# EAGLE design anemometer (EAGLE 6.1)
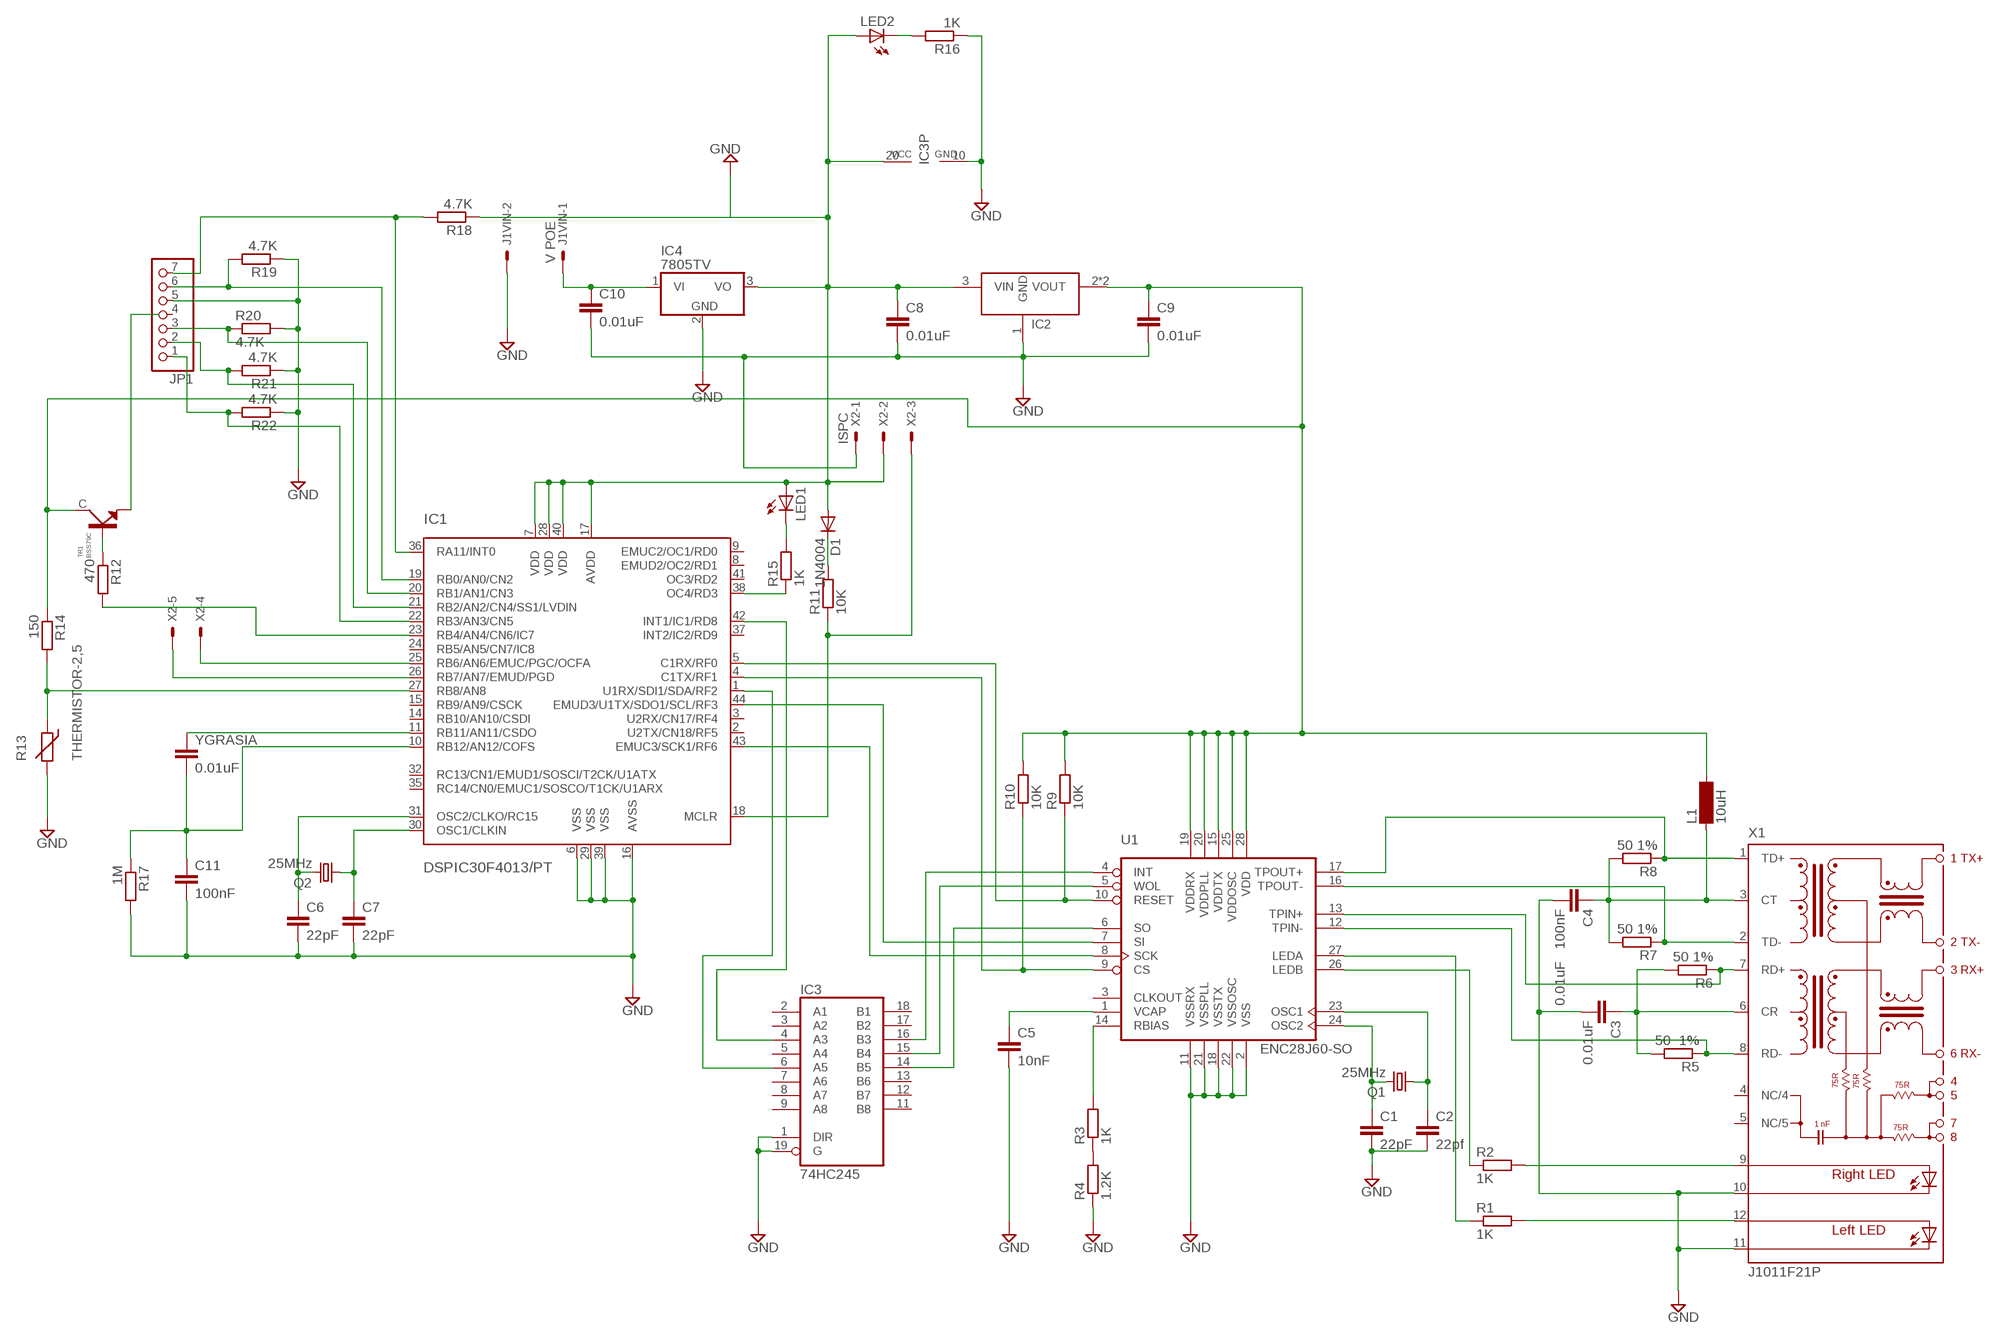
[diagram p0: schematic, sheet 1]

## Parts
C1  22pF  C-EUC0805  [C0805]
C2  22pf  C-EUC0805  [C0805]
C3  0.01uF  C-EUC0805  [C0805]
C4  0.01uF 100nF  C-EUC0805  [C0805]
C5  10nF  C-EU050-025X075  [C050-025X075]
C6  22pF  C-EUC0805  [C0805]
C7  22pF  C-EUC0805  [C0805]
C8  0.01uF  C-EU050-024X044  [C050-024X044]
C9  0.01uF  C-EU050-024X044  [C050-024X044]
C10  0.01uF  C-EU050-024X044  [C050-024X044]
C11  100nF  C-EUC0805  [C0805]
D1  1N4004  [DO41-10]
IC1  DSPIC30F4013/PT  [TQFP44]
IC2  TC2117-3.3  [SOT-223]
IC3  74HC245  [TSSOP20]
IC4  7805TV  [TO220V]
J1VIN  V POE  22-27-2021-02  [6410-02]
JP1  PINHD-1X7  [1X07]
L1  10uH  SM-1206  [SM-1206]
LED1  LEDSML0805  [SML0805]
LED2  LEDSML0805  [SML0805]
Q1  25MHz  CRYSTALHC49S  [HC49/S]
Q2  25MHz  CRYSTALHC49S  [HC49/S]
R1  1K  R-EU_R0805W  [R0805W]
R2  1K  R-EU_R0805W  [R0805W]
R3  1K  R-EU_R0805W  [R0805W]
R4  1.2K  R-EU_R0805W  [R0805W]
R5  50 1%  R-EU_R0603  [R0603]
R6  50 1%  R-EU_R0603  [R0603]
R7  50 1%  R-EU_R0603  [R0603]
R8  50 1%  R-EU_R0603  [R0603]
R9  10K  R-EU_R0805W  [R0805W]
R10  10K  R-EU_R0805W  [R0805W]
R11  10K  R-EU_R0805W  [R0805W]
R12  470  R-EU_R0805W  [R0805W]
R13  THERMISTOR-2,5  [RS-2,5]
R14  150  R-EU_R0805W  [R0805W]
R15  1K  R-EU_R0805W  [R0805W]
R16  1K  R-EU_R0805W  [R0805W]
R17  1M  R-EU_R0805W  [R0805W]
R18  4.7K  R-EU_R0805W  [R0805W]
R19  4.7K  R-EU_R0805W  [R0805W]
R20  4.7K  R-EU_R0805W  [R0805W]
R21  4.7K  R-EU_R0805W  [R0805W]
R22  4.7K  R-EU_R0805W  [R0805W]
TR1  BSS79C  [SOT23-EBC]
U1  ENC28J60-SO  [SO28W]
X1  J1011F21P  [J1]
X2  ISPC  22-23-2051  [22-23-2051]
YGRASIA  0.01uF  C-EU050-024X044  [C050-024X044]

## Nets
GND: C1.2 C2.2 C3.2 C4.2 C5.2 C6.2 C7.2 C8.2 C9.2 C10.2 C11.2 IC1.6(VSS) IC1.16(AVSS) IC1.29(VSS) IC1.39(VSS) IC2.1(GND) IC3.1(DIR) IC3.10(GND) IC3.19(G) IC4.2(GND) J1VIN.2 JP1.5 R4.1 R13.2 R16.1 R17.2 R19.1 R20.2 R21.1 R22.1 U1.2(VSS) U1.11(VSSRX) U1.18(VSSTX) U1.21(VSSPLL) U1.22(VSSOSC) X1.10(C-R) X1.11(C-L) X2.1
N$1: C1.1 Q1.2 U1.24(OSC2)
N$2: C2.1 Q1.1 U1.23(OSC1)
N$3: R1.1 U1.27(LEDA)
N$4: R1.2 X1.12(AL)
N$5: R2.1 U1.26(LEDB)
N$6: R2.2 X1.9(A-R)
N$7: R3.1 R4.2
N$8: R3.2 U1.14(RBIAS)
N$9: R6.1 U1.13(TPIN+) X1.7(RD+)
N$10: R5.1 U1.12(TPIN-) X1.8(RD-)
N$11: C3.1 R5.2 R6.2 X1.6(CR)
N$12: C6.1 IC1.31(OSC2/CLKO/RC15) Q2.2
N$13: R7.1 U1.16(TPOUT-) X1.2(TD-)
N$14: R8.1 U1.17(TPOUT+) X1.1(TD+)
N$15: C4.1 L1.1 R7.2 R8.2 X1.3(CT)
N$16: C7.1 IC1.30(OSC1/CLKIN) Q2.1
N$17: C5.1 U1.1(VCAP)
N$18: IC1.5(C1RX/RF0) R9.1 U1.10(RESET)
N$19: IC1.4(C1TX/RF1) R10.1 U1.9(CS)
N$20: IC1.18(MCLR) R11.1 X2.3
N$21: C10.1 IC4.1(VI) J1VIN.1
N$22: D1.C R11.2
N$23: C9.1 IC2.2(VOUT) IC2.4(VOUT) L1.2 R9.2 R10.2 R14.1 TR1.C U1.15(VDDTX) U1.19(VDDRX) U1.20(VDDPLL) U1.25(VDDOSC) U1.28(VDD)
N$24: IC3.14(B5) U1.6(SO)
N$25: C8.1 D1.A IC1.7(VDD) IC1.17(AVDD) IC1.28(VDD) IC1.40(VDD) IC2.3(VIN) IC3.20(VCC) IC4.3(VO) LED1.A LED2.A R18.1 X2.2
N$26: IC3.15(B4) U1.5(WOL)
N$27: IC3.16(B3) U1.4(INT)
N$28: IC1.26(RB7/AN7/EMUD/PGD) X2.5
N$29: IC1.25(RB6/AN6/EMUC/PGC/OCFA) X2.4
N$30: IC1.1(U1RX/SDI1/SDA/RF2) IC3.6(A5)
N$31: IC1.44(EMUD3/U1TX/SDO1/SCL/RF3) U1.7(SI)
N$32: IC1.43(EMUC3/SCK1/RF6) U1.8(SCK)
N$33: IC1.42(INT1/IC1/RD8) IC3.4(A3)
N$35: IC1.36(RA11/INT0) JP1.7 R18.2
N$36: IC1.19(RB0/AN0/CN2) JP1.6 R19.2
N$37: IC1.21(RB2/AN2/CN4/SS1/LVDIN) JP1.2 R21.2
N$38: TR1.E
N$39: IC1.22(RB3/AN3/CN5) JP1.1 R22.2
N$40: R12.1 TR1.B
N$41: IC1.23(RB4/AN4/CN6/IC7) R12.2
N$42: IC1.27(RB8/AN8) R13.1 R14.2
N$43: IC1.38(OC4/RD3) R15.1
N$44: LED1.C R15.2
N$45: LED2.C R16.2
N$46: IC1.20(RB1/AN1/CN3) JP1.3 R20.1
N$47: C11.1 IC1.10(RB12/AN12/COFS) R17.1 YGRASIA.2
N$53: IC1.11(RB11/AN11/CSDO) YGRASIA.1
Unconnected: IC1.2(U2TX/CN18/RF5) IC1.3(U2RX/CN17/RF4) IC1.8(EMUD2/OC2/RD1) IC1.9(EMUC2/OC1/RD0) IC1.14(RB10/AN10/CSDI) IC1.15(RB9/AN9/CSCK) IC1.24(RB5/AN5/CN7/IC8) IC1.32(RC13/CN1/EMUD1/SOSCI/T2CK/U1ATX) IC1.35(RC14/CN0/EMUC1/SOSCO/T1CK/U1ARX) IC1.37(INT2/IC2/RD9) IC1.41(OC3/RD2) IC3.2(A1) IC3.3(A2) IC3.5(A4) IC3.7(A6) IC3.8(A7) IC3.9(A8) IC3.11(B8) IC3.12(B7) IC3.13(B6) IC3.17(B2) IC3.18(B1) JP1.4 U1.3(CLKOUT) X1.4(NC/4) X1.5(NC/5)

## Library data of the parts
C1-C11 YGRASIA = rcl:C-EU: CAPACITOR, European symbol
D1 = diode:1N4004: DIODE
IC1 = microchip-dspic:DSPIC30F4013: dsPIC General DSP with CAN and I2S ports
IC2 = myLib:TC2117-3.3: TC2117-3.3 Microchip regulator at 3.3 V in SOT-223
IC3 = my74xx-eu:74*245: Octal BUS TRANSCEIVER, 3-state
IC4 = linear:78*: Positive VOLTAGE REGULATOR Source: http://cache.national.com/ds/LM/LM78L05.pdf http://www.fairchildsemi.com/ds/LM/LM7805.pdf
J1VIN = con-molex:22-?-02: CONNECTOR; OC_FARNELL: unknown; OC_NEWARK: unknown
JP1 = pinhead:PINHD-1X7: PIN HEADER
L1 = inductor-neosid:SM-1206: INDUCTOR; OC_FARNELL: unknown; OC_NEWARK: unknown
LED1 LED2 = led:LED: LED
Q1 Q2 = crystal:CRYSTAL: CRYSTAL; OC_FARNELL: 1667008; OC_NEWARK: unknown
R1-R12 R14-R22 = rcl:R-EU_: RESISTOR, European symbol
R13 = varistor:THERMISTOR: THERMISTOR
TR1 = myLib-5-XX:BSS79C: BSS79C NPN transistor in Sot-23
U1 = microchip-enc28j60:ENC28J60-*: Microchip 10Mbit Eth. contoller with SPI interface
X1 = con-pulse:J1011F: PULSEJACK (TM) 1x1 Tab-UP RJ45 10/100 Base-TX RJ45 1x1 Tab-UP with LEDs 8-pin (J1 series) and 6-pin (JP series) integrated magnetics connector, designed to support applications, such as ADSL modems, LAN-on-Motherboard, and Hub and Switches. Source: www.pulseeng.com .. PulseJack-J402.pdf; OC_FARNELL: unknown; OC_NEWARK: unknown
X2 = con-molex:22-23-2051: .100" (2.54mm) Center Header - 5 Pin; MF: MOLEX; MPN: 22-23-2051; OC_FARNELL: 1462952; OC_NEWARK: 38C9178

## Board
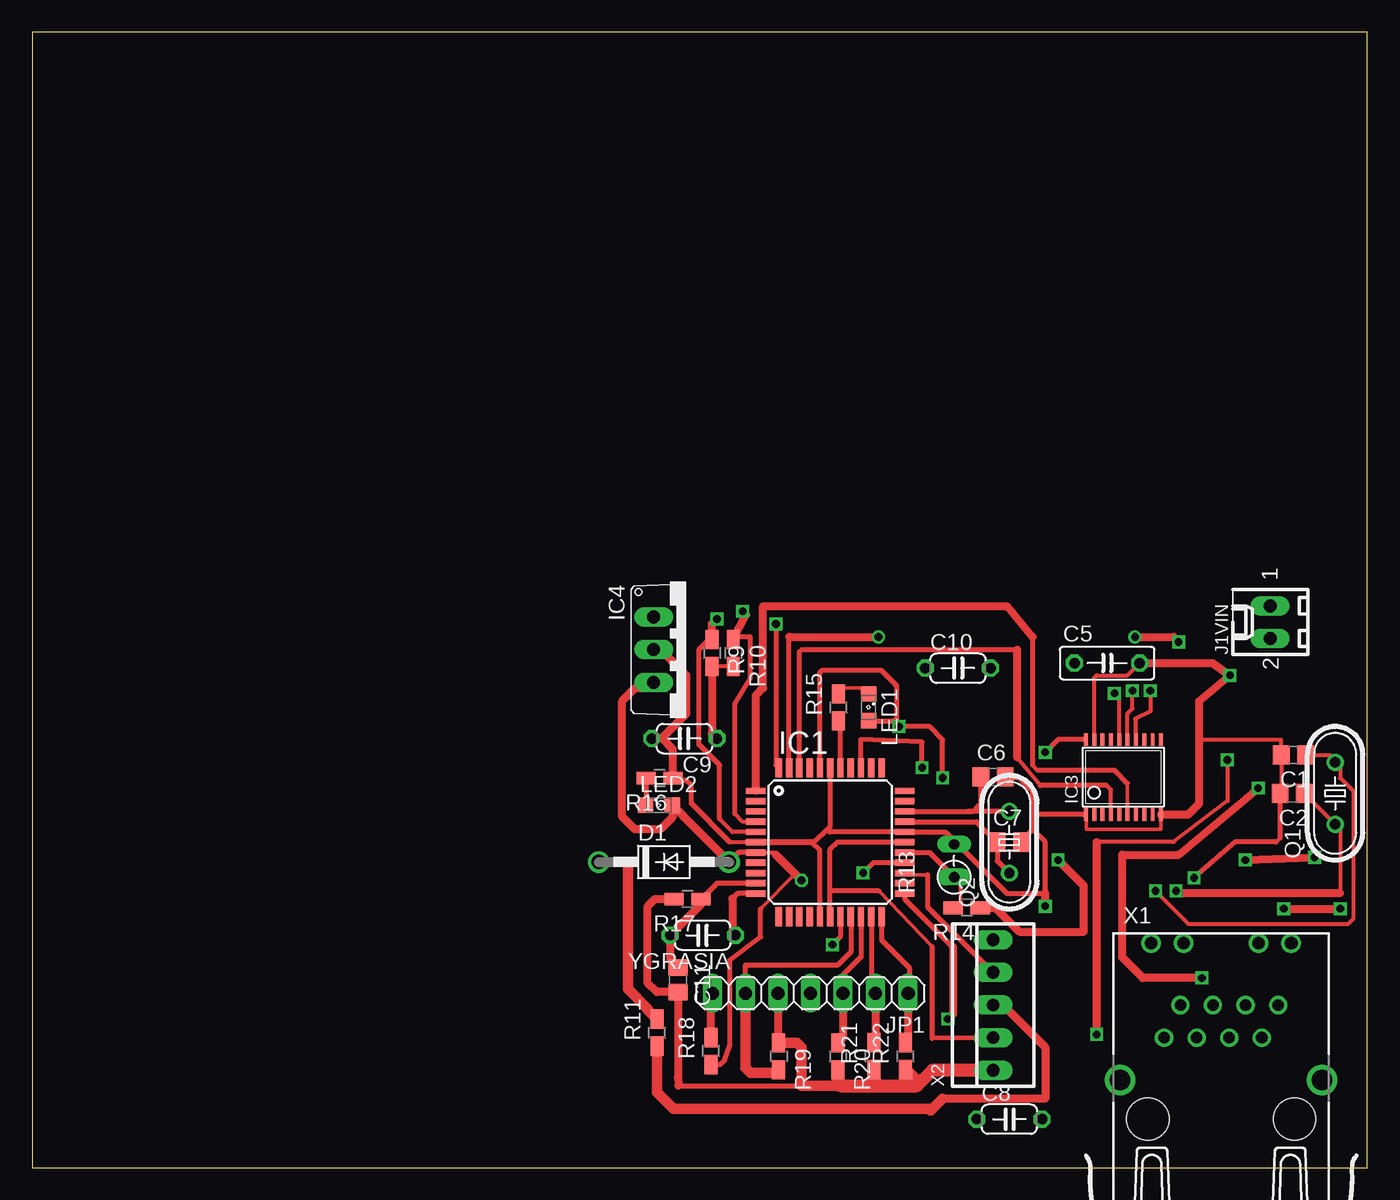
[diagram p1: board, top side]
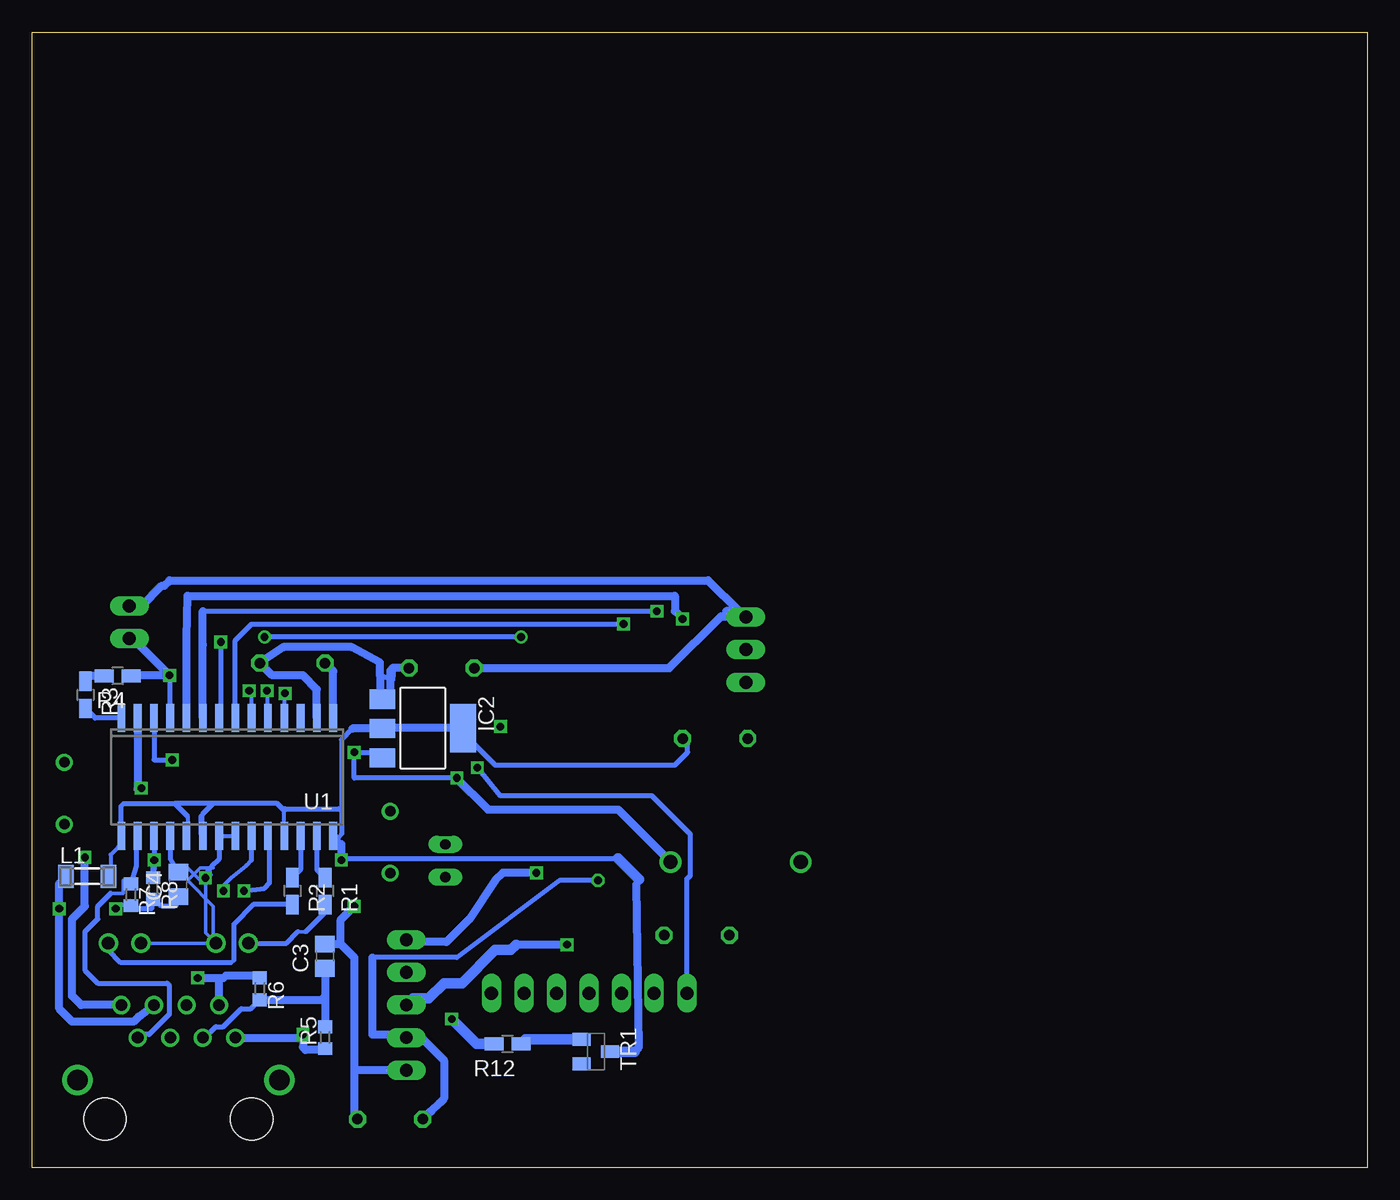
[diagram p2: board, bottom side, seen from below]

Size 104.12 x 88.57 mm. Coordinates in mm from the lower left corner, seen from the top.
Outline: 0,0 104.12,0 104.12,88.57 0,88.57 0,0
Copper layers (1*16): Top 0.035mm / dielectric 1.5mm / Bottom 0.035mm
Design rules: minimum track width 10mil, minimum drill 24mil, track to track 8mil, track to pad 8mil, pad to pad 8mil, via to via 8mil, smd to smd 8mil, copper to edge 40mil, drill to drill 8mil, minimum pad ring 10mil, minimum via ring 8mil, stop-mask expansion 4mil, vias tented up to drill 0mil, thermal gap 10mil

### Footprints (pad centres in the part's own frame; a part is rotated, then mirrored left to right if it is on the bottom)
C0805 = smd 1.3 x 1.5: 1 -0.95,0; 2 0.95,0
C050-025X075 = drill 0.813 octagon: 1 -2.54,0; 2 2.54,0
C050-024X044 = drill 0.813 octagon: 1 -2.54,0; 2 2.54,0
DO41-10 = drill 1.118: A 5.08,0; C -5.08,0
TQFP44 = smd 1.5 x 0.5: 1 -5.8,4; 2 -5.8,3.2; 3 -5.8,2.4; 4 -5.8,1.6; 5 -5.8,0.8; 6 -5.8,0; 7 -5.8,-0.8; 8 -5.8,-1.6; 9 -5.8,-2.4; 10 -5.8,-3.2; 11 -5.8,-4; 23 5.8,-4; 24 5.8,-3.2; 25 5.8,-2.4; 26 5.8,-1.6; 27 5.8,-0.8; 28 5.8,0; 29 5.8,0.8; 30 5.8,1.6; 31 5.8,2.4; 32 5.8,3.2; 33 5.8,4 | smd 0.5 x 1.5: 12 -4,-5.8; 13 -3.2,-5.8; 14 -2.4,-5.8; 15 -1.6,-5.8; 16 -0.8,-5.8; 17 0,-5.8; 18 0.8,-5.8; 19 1.6,-5.8; 20 2.4,-5.8; 21 3.2,-5.8; 22 4,-5.8; 34 4,5.8; 35 3.2,5.8; 36 2.4,5.8; 37 1.6,5.8; 38 0.8,5.8; 39 0,5.8; 40 -0.8,5.8; 41 -1.6,5.8; 42 -2.4,5.8; 43 -3.2,5.8; 44 -4,5.8
SOT-223 = smd 1.499 x 2.007: 1 -2.261,-3.15; 2 0.025,-3.15; 3 2.311,-3.15 | smd 3.81 x 2.007: 4 0,3.15
TSSOP20 = smd 0.305 x 0.991: 1 -2.925,-2.918; 2 -2.275,-2.918; 3 -1.625,-2.918; 4 -0.975,-2.918; 5 -0.325,-2.918; 6 0.325,-2.918; 7 0.975,-2.918; 8 1.625,-2.918; 9 2.275,-2.918; 10 2.925,-2.918; 11 2.925,2.918; 12 2.275,2.918; 13 1.625,2.918; 14 0.975,2.918; 15 0.325,2.918; 16 -0.325,2.918; 17 -0.975,2.918; 18 -1.625,2.918; 19 -2.275,2.918; 20 -2.925,2.918
TO220V = drill 1.016 long: 1 -2.54,-2.54; 2 0,-2.54; 3 2.54,-2.54
6410-02 = drill 1.016 long: 1 1.27,0; 2 -1.27,0
1X07 = drill 1.016 long: 1 -7.62,0; 2 -5.08,0; 3 -2.54,0; 4 0,0; 5 2.54,0; 6 5.08,0; 7 7.62,0
SM-1206 = smd 1.2 x 1.8: 1 -1.65,0; 2 1.65,0
SML0805 = smd 1.2 x 1.2: A 1.05,0; C -1.05,0
HC49/S = drill 0.813: 1 -2.413,0; 2 2.413,0
R0805W = smd 1.5 x 1: 1 -1.052,0; 2 1.052,0
R0603 = smd 1 x 1.1: 1 -0.85,0; 2 0.85,0
RS-2,5 = drill 0.813 long: 1 -1.27,0; 2 1.27,0
SOT23-EBC = smd 1 x 1.4: B -0.95,-1.1; C 0,1.1; E 0.95,-1.1
SO28W = smd 0.6 x 2.2: 1 -8.255,-4.6; 2 -6.985,-4.6; 3 -5.715,-4.6; 4 -4.445,-4.6; 5 -3.175,-4.6; 6 -1.905,-4.6; 7 -0.635,-4.6; 8 0.635,-4.6; 9 1.905,-4.6; 10 3.175,-4.6; 11 4.445,-4.6; 12 5.715,-4.6; 13 6.985,-4.6; 14 8.255,-4.6; 15 8.255,4.6; 16 6.985,4.6; 17 5.715,4.6; 18 4.445,4.6; 19 3.175,4.6; 20 1.905,4.6; 21 0.635,4.6; 22 -0.635,4.6; 23 -1.905,4.6; 24 -3.175,4.6; 25 -4.445,4.6; 26 -5.715,4.6; 27 -6.985,4.6; 28 -8.255,4.6
J1 = drill 0.9 pad 1.3: 1 4.445,2.54; 2 3.175,0; 3 1.905,2.54; 4 0.635,0; 5 -0.635,2.54; 6 -1.905,0; 7 -3.175,2.54; 8 -4.445,0 | drill 1 pad 1.422: 9 5.465,7.37; 10 2.925,7.37; 11 -2.925,7.37; 12 -5.465,7.37 | drill 1.6 pad 2.184: M1 -7.875,-3.3; M2 7.875,-3.3 | hole 3.3: 5.715,-6.35; -5.715,-6.35
22-23-2051 = drill 1 long: 1 -5.08,0; 2 -2.54,0; 3 0,0; 4 2.54,0; 5 5.08,0

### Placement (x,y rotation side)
C1  98.35,32.2 180 top
C2  98.25,29.21 180 top
C3  81.28,16.51 90 bottom
C4  92.71,22.11 90 bottom
C5  83.82,39.37 0 top
C6  74.93,30.48 0 top
C7  76.2,25.4 0 top
C8  76.2,3.81 0 top
C9  50.86,33.48 180 top
C10  72.19,38.97 0 top
C11  50.36,14.67 270 top
D1  49.26,23.86 0 top
IC1  62.23,25.4 0 top
IC2  73.66,34.29 270 bottom
IC3  85.09,30.48 0 top
IC4  51,40.41 270 top
J1VIN  96.53,42.56 90 top
JP1  60.69,13.62 180 top
L1  99.82,22.74 0 bottom
LED1  65.22,35.91 270 top
LED2  48.88,28.29 0 top
Q1  101.6,29.21 90 top
Q2  76.2,25.4 90 top
R1  81.28,21.59 270 bottom
R2  83.82,21.59 270 bottom
R3  99.96,36.89 270 bottom
R4  97.44,38.37 180 bottom
R5  81.28,10.16 90 bottom
R6  86.36,13.97 270 bottom
R7  96.41,21.3 270 bottom
R8  94.67,21.78 270 bottom
R9  53.01,40.15 270 top
R10  54.67,40.15 270 top
R11  48.73,10.55 90 top
R12  67.04,9.67 180 bottom
R13  71.88,23.96 90 top
R14  72.88,20.29 180 top
R15  62.88,35.91 90 top
R16  48.92,30.39 180 top
R17  51.11,20.96 180 top
R18  52.93,9.12 90 top
R19  58.21,8.7 270 top
R20  62.83,8.7 270 top
R21  65.63,8.72 90 top
R22  68.09,8.72 90 top
TR1  60.16,9.07 270 bottom
U1  88.9,30.48 180 bottom
X1  92.71,10.16 0 top
X2  74.93,12.7 90 top
YGRASIA  52.29,18.15 180 top

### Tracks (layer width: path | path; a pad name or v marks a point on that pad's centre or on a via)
GND  (via drill 0.6)
  Top 0.254: 48,33.41 C9.2 | IC3.10 88.02,26.43 88,26.41 82.2,26.41 82.2,27.53 IC3.1
  Top 0.305: IC3.19 82.81,38.22 83,38.41 85.4,38.41 C5.2 86.04,39.37 86,39.41 | 97.3,25.71 97,25.41 | C2.2 97.4,29.31 C1.2 97.4,33.41 91,33.41 | IC1.6 54.41,25.4 | 50.15,30.21 R16.1 | 49.1,33.51 49,33.61 48.2,33.61 48,33.41
  Top 0.406: C2.2 97.3,25.71 | 97,25.41 93.8,25.41 v90.6,22.61 | IC1.39 62.23,26.64 62,26.41 | 62,26.41 61,25.41 IC1.6 60.81,25.4 61.43,24.78 IC1.16 | 62,26.41 62.21,26.2 IC1.29 71.21,26.2 72,25.41 | C7.2 77.15,25.56 78,26.41 | 78,26.41 78,27.41 | 78,27.41 78,29.41 77,30.41 75.95,30.41 C6.2 | R13.2 71.88,25.29 72,25.41 | 72,25.41 76,21.41 79,21.41 79,25.41 78,26.41 | IC3.1 78.15,27.56 78,27.41 | 58.15,9.81 R19.1 | 50.4,6.41 60,6.41 | R16.1 50.18,30.39 | 54.41,25.4 51.4,28.41 51.4,29.81 51,30.21 50.15,30.21
  Top 0.61: IC3.10 90.15,27.56 91,28.41 91,33.41 91,36.41 v93.4,38.41 92.04,39.37 C5.2 | v79,20.41 79,21.41 | JP1.5 58.15,9.81 | 50.4,6.41 50.36,7.05 C11.2 48.69,13.72 48,14.41 48,20.41 48.55,20.96 R17.2 | R16.1 49.97,32.64 49.1,33.51 51,35.41 51,38.41 49,40.41 IC4.2
  Top 0.813: R19.1 59.66,9.75 60,9.41 60,6.41 62.66,6.41 62.83,6.58
  Top 1.016: X2.1 70.21,7.62 69,6.41 | 69,6.41 69,6.76 R22.1 | R20.2 62.83,6.58 63,6.41 66,6.41 | 66,6.41 69,6.41 | R21.1 65.63,6.78 66,6.41
  Bottom 0.254: 76.2,38.77 76.12,38.09 | 90.17,22.86 v90.6,22.61 | 92.71,22.86 C4.2 | 76.2,36.83 IC2.1 | 48,33.41 C9.2 | X1.10 X1.11 | v90.6,22.61 90.6,18.35 X1.11 | 93,23.41 C4.2 | C4.2 92,23.41 91,22.41 v90.6,22.61 | X1.11 90,17.41 90,20.41 92,22.41 91,23.41 90,23.41 90.1,23.51
  Bottom 0.305: 92.4,23.21 92.6,23.41 93,23.41 | U1.21 U1.22
  Bottom 0.406: 76.12,38.09 77,38.41 | U1.18 93.34,24.1 C4.2 | U1.21 89.53,24.07 90.1,23.51 90.4,23.21 | 96.35,38.41 R4.1 | U1.11 93.34,38.06 v93.4,38.41
  Bottom 0.61: C10.2 76.04,38.97 76.12,38.09 | 77,36.41 77,38.41 77,39.41 79.2,40.61 84.52,40.61 C5.2 85.4,38.41 83,38.41 81.92,37.33 U1.2 | 96.35,38.41 v93.4,38.41 96.28,41.29 J1VIN.2 | X2.1 78.79,7.62 79,7.41 | 79,7.41 79,4.07 C8.2 | C3.2 80.05,17.46 | 80.05,17.46 79,16.41 79,7.41 | 80.05,17.46 80.05,19.36 v79,20.41 | 76.2,38.77 76.2,36.83
N$1  (via drill 0.6)
  Top 0.305: Q1.2 101.79,31.62 | 101.79,31.62 102,31.41 102,30.41 103,29.41 103,19.41 102.6,19.01 90.2,19.01 v87.6,21.61 87.8,21.61 88,21.41 | C1.1 101.21,32.2 101.79,31.62
  Bottom 0.305: 85.6,25.75 U1.24
  Bottom 0.406: v87.6,21.61 86,21.81 85.6,22.21 85.6,25.75
N$2  (via drill 0.6)
  Top 0.305: Q1.1 99.19,29.21 C2.1 102,26.41 102,21.41 | 89.6,21.41 v89.2,21.61
  Top 0.61: 102,21.41 89.6,21.41
  Bottom 0.305: U1.23 87,25.42 87,25.41 87,25.61 | v89.2,21.61 89.4,21.81 88.6,22.61 87.4,23.61 87,24.01
  Bottom 0.406: 87,24.01 87,25.41
N$3
  Bottom 0.406: U1.27 81.92,23.28 R1.1
N$4
  Bottom 0.254: 83.4,18.41 82.8,18.41 | 81.2,20.01 81.2,20.46 R1.2
  Bottom 0.406: X1.12 84.28,17.53 83.4,18.41 | 82.8,18.41 81.2,20.01
N$5
  Bottom 0.406: U1.26 83.19,23.28 R2.1
N$6
  Bottom 0.254: 88.4,16.21 88.6,16.01 | 98.2,17.01 98.2,17.5 X1.9
  Bottom 0.406: R2.2 86.87,20.54 88.4,19.01 88.4,16.21 | 88.6,16.01 97.2,16.01 98.2,17.01
N$7
  Bottom 0.406: 99.96,38.37 100,38.41 100,37.98 R3.1
  Bottom 0.61: R4.2 99.96,38.37
N$8
  Bottom 0.406: U1.14 99.2,35.08 R3.2
N$9  (via drill 0.6)
  Top 0.61: v91.2,14.81 86.6,14.81 85,16.41 85,24.41 89.4,24.41 v95.6,29.61
  Bottom 0.305: 89.53,14.68 89.2,15.01 89,15.01 89.2,14.81 | 86.55,15.01 R6.1 | 96,29.41 95.89,29.53 95.69,29.53 v95.6,29.61
  Bottom 0.61: X1.7 89.53,14.68 | 89,15.01 86.55,15.01 | v91.2,14.81 89.2,14.81 | U1.13 95.89,29.53
N$10  (via drill 0.6)
  Top 0.305: v93.2,31.81 93.2,28.61 89,25.41 83,25.41
  Top 0.61: 83,25.41 v83,10.41
  Bottom 0.305: X1.8 86.55,10.16 | 81.38,9.21 R5.1 | 83.25,10.16 v83,10.41
  Bottom 0.406: U1.12 94.61,31.82 v93.2,31.81
  Bottom 0.61: v83,10.41 83,9.41 82.8,9.21 81.38,9.21 | X1.8 83.25,10.16
N$11
  Bottom 0.305: X1.6 90.65,10.16 | 81.57,13.12 81.28,13.41
  Bottom 0.406: 90.65,10.16 89.8,11.01 89.2,11.01 87.8,12.41 87.07,12.41 R6.2
  Bottom 0.61: C3.1 81.28,13.41 R5.2 | R6.2 81.57,13.12
N$12
  Top 0.406: IC1.31 73,27.8 | 73,27.8 73.39,27.8 74,28.41 74,30.46 C6.1 | Q2.2 73.01,27.81 73,27.8
N$13
  Bottom 0.254: 98,21.41 97,21.41 97,22.41 96,22.41 R7.1
  Bottom 0.305: U1.16 95.89,25.53 96,25.41
  Bottom 0.406: 96,25.41 96,23.56 R7.1 | X1.2 95.64,10.41 95,10.41 93.4,12.01 93.4,14.21 93.6,14.41 99,14.41 100,15.41 100,18.41 99,19.41 99,20.41 98,21.41
N$14  (via drill 0.6)
  Top 0.305: 99.8,24.21 v100,24.21
  Top 0.61: v94.6,24.01 99.8,24.21
  Bottom 0.305: 94.61,23.29 R8.1 | 94.67,24.14 v94.6,24.01
  Bottom 0.406: U1.17 94.61,23.29 | R8.1 94.67,24.14
  Bottom 0.61: X1.1 100.29,12.7 101,13.41 101,19.41 100,20.41 v100,24.21
N$15  (via drill 0.6)
  Top 0.61: v97.6,20.21 v102,20.21
  Bottom 0.254: R8.2 95,21.41 95,20.41 94.8,20.41 | 96,20.21 96,20.41 R7.2
  Bottom 0.305: 102,22.21 L1.1 | 94.64,20.96 R8.2 | R7.2 96.41,20.82 v97.6,20.21
  Bottom 0.406: C4.1 92.71,20.7 93,20.41 94,20.41 94.6,21.01 94.8,21.01 94.8,20.41 94.8,20.21 96,20.21 96.2,20.41
  Bottom 0.61: X1.3 95.81,11.79 96.2,11.41 101,11.41 102,12.41 v102,20.21 102,22.21
N$16
  Top 0.406: IC1.30 73.65,27 C7.1 75.25,23.94 Q2.1
N$17
  Bottom 0.61: U1.1 80.64,38.73 C5.1
N$18  (via drill 0.6)
  Top 0.305: 53,42.41 53.01,42.4 R9.1 52.79,41.2 | IC1.5 54.61,26.2 53.6,27.21
  Top 0.406: 52.79,41.2 52,40.41 52,33.01 53.6,31.41 53.6,27.21
  Top 0.61: R9.1 53.01,42.42 v53.4,42.81
  Bottom 0.61: U1.10 92.08,41.33 92,44.61 54,44.61 54,43.41 v53.4,42.81
N$19  (via drill 0.6)
  Top 0.305: IC1.4 55.41,27 54.8,27.61 | 55.67,43.14 v55.4,43.41 | R10.1 54.79,41.2 55,41.41
  Top 0.406: 54.8,27.61 54.8,36.21 56,38.21 56,41.41 55,41.41
  Top 0.61: R10.1 55.67,43.14
  Bottom 0.406: 90.8,43.41 v55.4,43.41
  Bottom 0.61: U1.9 90.81,40.81 90.8,43.41
N$20  (via drill 0.6)
  Top 0.406: IC1.18 63.03,18.04 v62.4,17.41 | 70,4.61 70.1,4.51
  Top 0.61: X2.3 75.71,12.7 79,9.41 79,5.41 71,5.41 | 70.1,4.51 70,4.41
  Top 0.813: 71,5.41 70.1,4.51 | 70,4.61 50,4.61 48.73,5.88 R11.1
  Bottom 0.406: 74.42,13.21 X2.3
  Bottom 0.61: v62.4,17.41 66.4,17.41
  Bottom 0.813: 74.42,13.21 73.2,13.21 72,14.41 70.6,14.41 68,17.01 66.8,17.01 66.4,17.41
N$21
  Bottom 0.254: 49,43.41 IC4.1
  Bottom 0.61: C10.1 54.44,38.97 50.4,43.01 48.52,43.01 IC4.1 | J1VIN.1 95.58,43.83 94,45.41 93.8,45.41 93.4,45.81 51.4,45.81 49,43.41 50,43.41
N$22
  Top 0.61: D1.C 46.45,23.86
  Top 0.813: 46.45,23.86 46.45,13.96 48,12.41 48,12.33 R11.2
N$23  (via drill 0.6)
  Top 0.305: R10.2 R9.2
  Top 0.61: R9.2 53.01,33.87 C9.1 | R14.1 75.12,20.29 77,18.41 82,18.41 82,22.01 v80,24.01
  Bottom 0.254: 80.01,24.13 v80,24.01
  Bottom 0.305: 80,26.01 80.17,25.81 U1.28 | 84.4,28.01 84.45,27.96 U1.25 84.45,27.86 | 80.2,28.01 80,27.81 | 97.16,28.25 97,28.41 | 92,27.41 92,25.96 U1.19 | U1.15 97,25.72 97,25.41 98,24.41 98,22.91 L1.2 | 90.81,27.61 91,27.41 91,26.07 U1.20 90.81,27.61
  Bottom 0.406: 79.14,34.27 80,33.41 80,27.81 80,26.01 | 84.4,28.01 80.2,28.01 | 84.45,27.86 85,28.41 90,28.41 | U1.15 97.16,28.25 | 97,28.41 93,28.41 | 93,28.41 92,27.41 | 90.81,27.61 90,28.41 | 90,28.41 93,28.41 | IC2.4 70.51,33.92 68,31.41 54,31.41 53,32.41 53,33.08 C9.1 | 76.88,34.29 77,34.41 76.95,34.41 IC2.2 | 80,25.24 U1.28 | 80.01,24.13 58.42,24.13
  Bottom 0.61: IC2.2 79.14,34.27 | IC2.4 76.88,34.29 | v80,24.01 80,25.24 | 57.14,9.07 56.8,9.41 57,22.11 56.8,22.51
  Bottom 0.813: TR1.C 57.14,9.07 | 56.8,22.51 58.42,24.13
N$24  (via drill 0.6)
  Top 0.305: v87.2,37.21 87.2,35.61 86,35.01 86.06,34.94 IC3.14
  Bottom 0.305: U1.6 87,37 v87.2,37.21
N$25  (via drill 0.6, 0.61)
  Top 0.254: 70.19,17.24 66.04,21.59 | 56.8,20.21 59.5,22.91
  Top 0.305: IC1.7 57.81,24.6 58,24.41
  Top 0.406: IC3.20 79.99,33.4 v79,32.41 | IC1.28 62.79,25.4 62.23,24.84 62.23,21.59 | IC1.17 62.23,21.59 | IC1.40 61.43,38.64 61.6,38.81 66.2,38.81 67.4,37.61 67.4,34.61 v67.6,34.41 | LED1.A 67.15,34.86 v67.6,34.41 | IC1.7 55.08,24.6 D1.A | 66.04,21.59 62.23,21.59 | 70.19,17.24 70.19,10.1 X2.2 | v71,30.41 71,33.41 70,34.41 v67.6,34.41 | R18.1 53.66,8.07 54,8.41 54.4,9.61 54.4,16.21 56.8,18.01 56.8,20.21
  Top 0.61: D1.A 50.79,27.41 50.79,27.43 LED2.A 49.93,27.34 49,26.41 47,26.41 46,27.41 46,36.41 47,37.41 48,37.41 IC4.3 | 58,24.41 59.5,22.91 v60,22.41
  Bottom 0.254: 71.12,30.48 v71,30.41 | 54.61,24.13 D1.A | 72.39,5.08 72.36,5.05 | 75,10.41 X2.2
  Bottom 0.305: 77.24,32.41 IC2.3
  Bottom 0.406: 77.24,32.41 v79,32.41 79,30.41 v71,30.41 | 77.6,16.41 71,16.41 63,22.41 v60,22.41
  Bottom 0.61: X2.2 73.75,10.16 72,8.41 72,5.41 72.36,5.05 73,4.41 73.06,4.41 C8.1 | 54.61,24.13 58.42,27.94 68.58,27.94 71.12,30.48 | 75,10.41 77.6,10.41 77.6,16.41
N$26  (via drill 0.6)
  Top 0.305: IC3.15 85.42,35.42 85.8,35.81 v85.8,37.21
  Bottom 0.305: v85.8,37.21 85.8,35.16 U1.5
N$27  (via drill 0.6)
  Top 0.305: IC3.16 84.77,36.84 v84.4,37.01
  Bottom 0.305: v84.4,37.01 84.6,35.22 U1.4
N$28  (via drill 0.6)
  Top 0.406: IC1.26 65.59,23.8 v64.8,23.01
  Bottom 0.406: 75.4,17.61 75.1,17.61 X2.5
  Bottom 0.61: v64.8,23.01 67.4,23.01 68,22.41 70,19.41 71.8,17.61 75.1,17.61
N$29
  Top 0.254: 69.85,22.86 68.58,22.86 IC1.25
  Top 0.406: 69.85,22.86 69.85,20.32 X2.4
N$30
  Top 0.254: IC3.6 85.42,30
  Top 0.305: 84.77,30.64 84.5,30.91 84.4,31.01 | 78.4,31.01 78,31.41
  Top 0.406: 78,41.41 78,31.41 | 84.4,31.01 78.4,31.01 | 85.42,30 84.5,30.91
  Top 0.61: IC1.1 56.43,36.84 57,37.41 57,43.81 76,43.81 78,41.41
N$31  (via drill 0.6)
  Top 0.254: 58,31.41 IC1.44
  Top 0.406: v58,42.41 58,31.41
  Bottom 0.406: U1.7 88.27,41.14 87,42.41 v58,42.41
N$32  (via drill 0.6, 0.61)
  Top 0.254: 89,41.41 v89.4,41.01 | 59,41.41 59.03,41.41
  Top 0.305: 59.03,41.41 59.03,41.44
  Top 0.406: IC1.43 59.03,41.41
  Top 0.61: v86,41.41 89,41.41 | 59.03,41.41 v66,41.41
  Bottom 0.305: 89.4,35.22 U1.8
  Bottom 0.406: v89.4,41.01 89.4,35.22 | v66,41.41 v86,41.41
N$33
  Top 0.305: 59.83,40.24 60,40.41 | 76.8,32.01 78.6,29.81 | IC3.4 84.11,29.5 83.8,29.81
  Top 0.406: IC1.42 59.83,40.24 | 60,40.41 76.8,40.41 | 83.8,29.81 78.6,29.81
  Top 0.61: 76.8,40.41 76.8,32.01
N$35  (via drill 0.6)
  Top 0.254: 52.93,13.48 JP1.7
  Top 0.406: v69.4,31.21 69.4,33.21 64.6,33.41 64.6,31.23 IC1.36
  Top 0.61: R18.2 52.93,13.48
  Bottom 0.406: JP1.7 53.07,22.54 52.8,22.81 52.8,26.01 55.8,29.01 67.6,29.01 v69.4,31.21
N$36
  Top 0.406: IC1.19 63.83,16.84 62.8,15.81 55.6,15.81 JP1.6
  Top 0.813: JP1.6 55.61,7.8 56,7.41 57.97,7.41 R19.2
N$37
  Top 0.406: IC1.21 65.43,13.96 JP1.2 | 65.77,9.91 R21.2
  Top 0.61: JP1.2 65.77,9.91
N$39
  Top 0.406: IC1.22 66.23,17.78 68.4,15.61 68.4,13.71 JP1.1 | 68.31,9.99 R22.2
  Top 0.61: JP1.1 68.31,9.99
N$40
  Bottom 0.813: TR1.B 65.64,10.02 R12.1
N$41  (via drill 0.6)
  Top 0.406: IC1.23 68.03,20.98 71.8,17.21
  Top 0.61: 71.8,17.21 71.8,12.01 v71.4,11.61
  Bottom 0.813: R12.2 69.46,9.67 v71.4,11.61
N$42
  Top 0.254: R14.2 72.39,20.32 72.39,22.86 R13.1
  Top 0.406: IC1.27 69.97,24.6 R13.1
N$43
  Top 0.406: IC1.38 63.03,34.71 R15.1
N$44
  Top 0.254: LED1.C 65,37.41 63,37.41 R15.2
N$45
  Top 0.406: R16.2 47.87,28.33 LED2.C
N$46
  Top 0.406: IC1.20 64.63,16.44 63.2,15.01 63.2,13.65 JP1.3 | 63.23,10.15 R20.1
  Top 0.61: JP1.3 63.23,10.15
N$47
  Top 0.406: IC1.10 53.4,22.2 R17.1 52.16,20.56 | 49.75,16.23 C11.1
  Top 0.61: 52.16,20.56 YGRASIA.2 49.75,16.23
N$53
  Top 0.406: IC1.11 54.99,21.4 54.6,21.01
  Top 0.61: 54.6,21.01 54.6,18.38 YGRASIA.1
